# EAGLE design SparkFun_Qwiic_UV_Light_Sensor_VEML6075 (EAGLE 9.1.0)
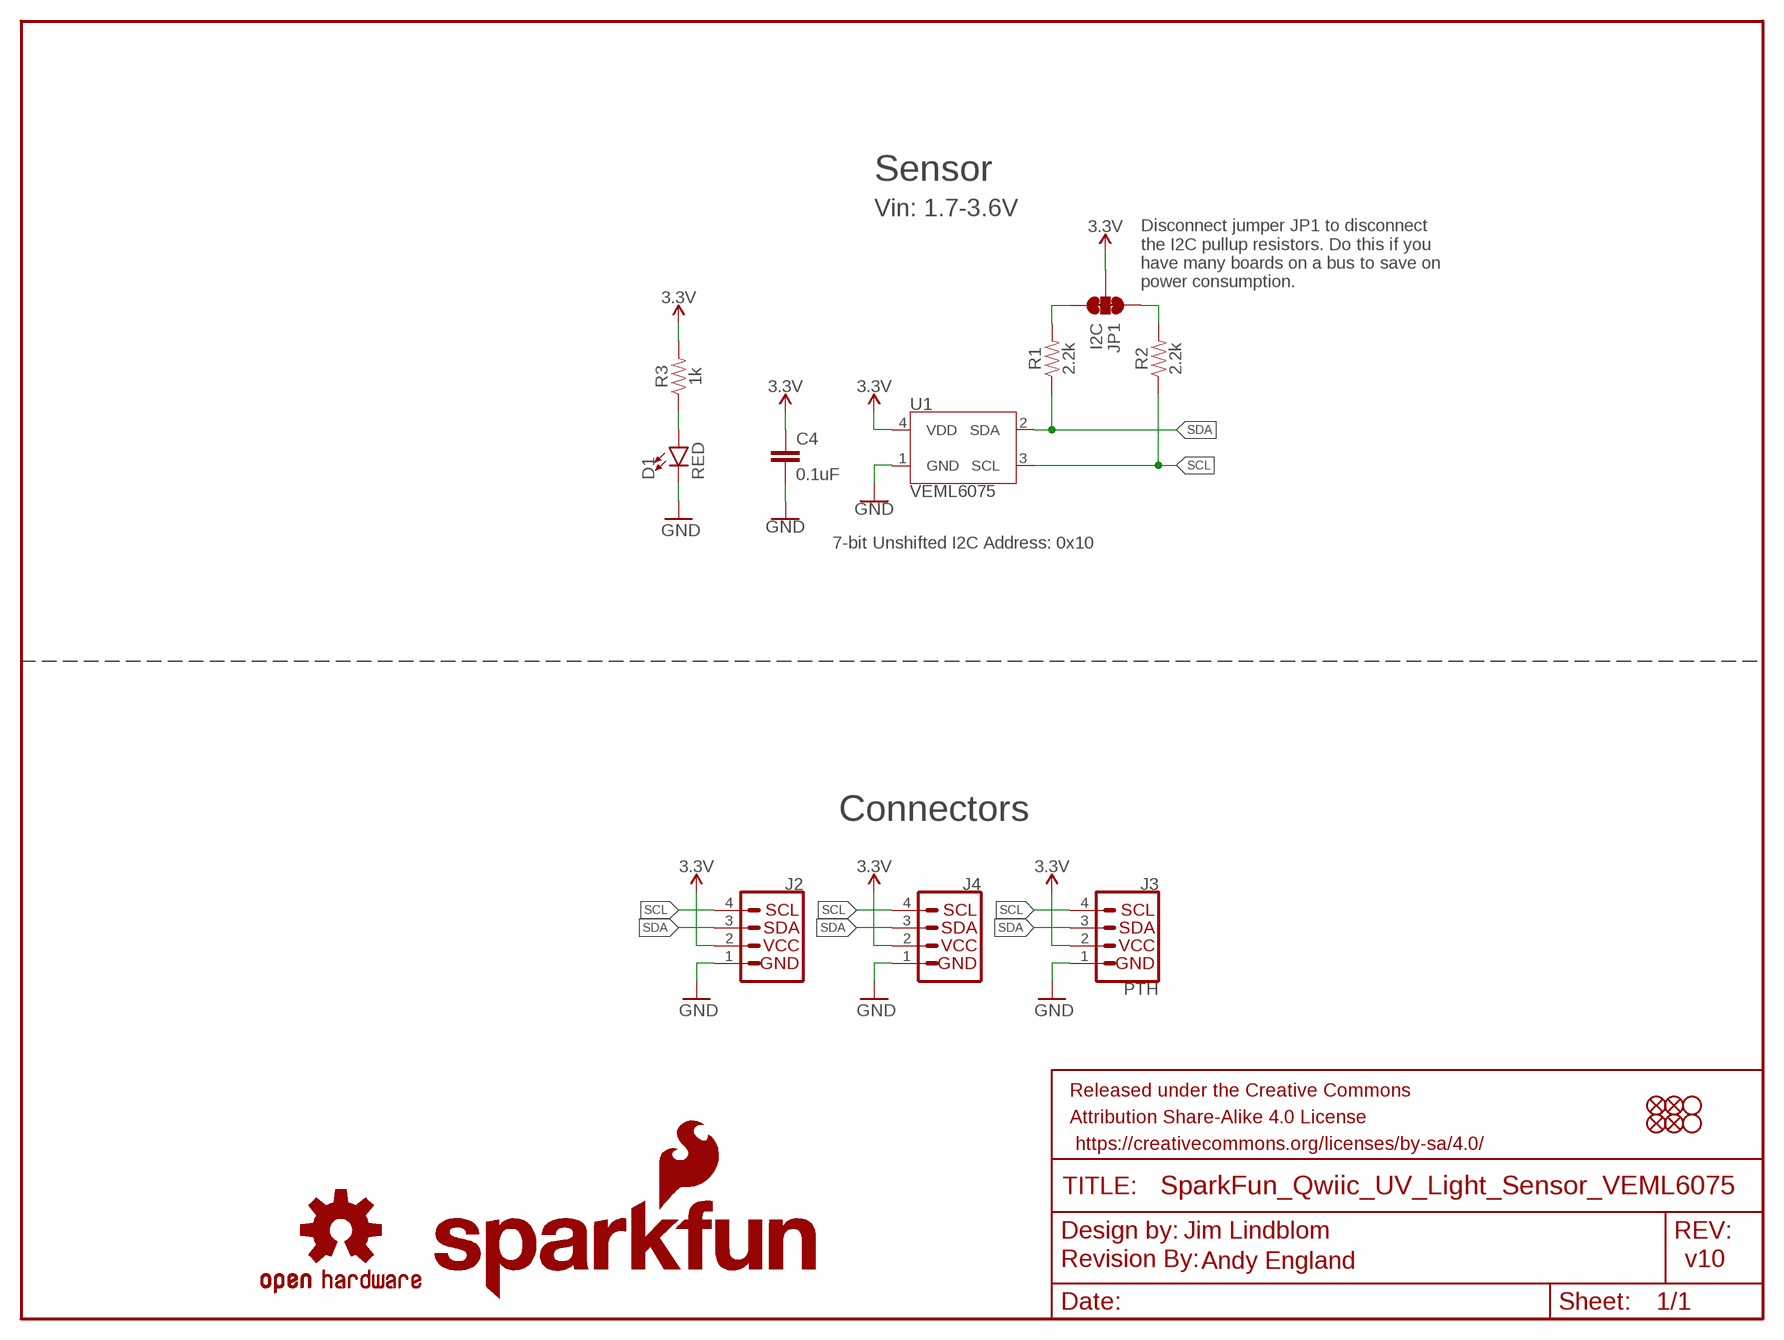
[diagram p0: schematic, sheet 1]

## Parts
C4  0.1uF  0.1UF-0603-25V-(+80/-20%)  [0603]
D1  RED  LED-RED0603  [LED-0603]
FRAME1  FRAME-LETTER  [CREATIVE_COMMONS]
J2  QWIIC_CONNECTORJS-1MM  [1X04_1MM_RA]
J3  PTH  I2C_STANDARD_NO_SILK  [1X04_NO_SILK]
J4  QWIIC_CONNECTORJS-1MM  [1X04_1MM_RA]
JP1  I2C  JUMPER-SMT_3_2-NC_TRACE_SILK  [SMT-JUMPER_3_2-NC_TRACE_SILK]
JP2  FIDUCIALUFIDUCIAL  [MICRO-FIDUCIAL]
JP3  STAND-OFF  [STAND-OFF]
JP4  STAND-OFF  [STAND-OFF]
JP5  FIDUCIALUFIDUCIAL  [MICRO-FIDUCIAL]
JP6  FIDUCIALUFIDUCIAL  [MICRO-FIDUCIAL]
JP7  FIDUCIALUFIDUCIAL  [MICRO-FIDUCIAL]
LOGO1  OSHW-LOGOMINI  [OSHW-LOGO-MINI]
LOGO2  REVISION  [REVISION]
R1  2.2k  2.2KOHM-0603-1/10W-1%  [0603]
R2  2.2k  2.2KOHM-0603-1/10W-1%  [0603]
R3  1k  1KOHM-0603-1/10W-1%  [0603]
U1  VEML6075  [VEML6075_A3OP]
U$1  SFE_LOGO_NAME_FLAME.1_INCH  [SFE_LOGO_NAME_FLAME_.1]
U$2  SFE_LOGO_NAME_FLAME.1_INCH  [SFE_LOGO_NAME_FLAME_.1]

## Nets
3.3V: C4.1 J2.2 J3.2(VCC) J4.2 JP1.2 R3.2 U1.4(VDD)
GND: C4.2 D1.C J2.1 J3.1(GND) J4.1 U1.1(GND)
N$3: D1.A R3.1
N$4: JP1.3 R1.2
N$5: JP1.1 R2.2
SCL: J2.4 J3.4(SCL) J4.4 R2.1 U1.3(SCL)
SDA: J2.3 J3.3(SDA) J4.3 R1.1 U1.2(SDA)

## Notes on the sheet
- Sensor
- Vin: 1.7-3.6V
- Disconnect jumper JP1 to disconnect 
  the I2C pullup resistors. Do this if you 
  have many boards on a bus to save on
  power consumption.
- 7-bit Unshifted I2C Address: 0x10
- Connectors
- Jim Lindblom
- Andy England | v10

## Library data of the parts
C4 = SparkFun-Capacitors:0.1UF: 0.1µF ceramic capacitors; PROD_ID: CAP-00810
D1 = SparkFun-LED:LED-RED: Red SMD LED; PROD_ID: DIO-00819
FRAME1 = SparkFun-Aesthetics:FRAME-LETTER: Schematic Frame - Letter
J2 J4 = SparkFun-Connectors:QWIIC_CONNECTOR: SparkFun I2C Standard Qwiic Connector An SMD 1mm pitch JST connector makes it easy and quick (get it? Qwiic?) to connect I2C devices to each other. The Qwiic system enables fast and solderless connection between popular platforms and various sensors and actuators. We carry 200mm, 100mm, 50mm, and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; PROD_ID: CONN-13694
J3 = SparkX:I2C_STANDARD: SparkFun I2C Standard Pinout Header SparkFun has standardized on a pinout for all I2C based sensor breakouts. This pinout allows I2C boards to be plugged directly into the headers on Arduino Uno compatible boards, and to be daisy chained easily. Example SparkFun Products: SparkFun Atmospheric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
JP1 = SparkFun-Jumpers:JUMPER-SMT_3_2-NC_TRACE: Normally closed trace jumper (2 of 2 connections) This jumper has a trace between all three pads so they are normally closed (NC). Use a razor knife to open the connection(s). For best results follow the IPC guidelines for cutting traces: Cutout at least 0.063 mm (0.005 in). Remove all loose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
JP2 JP5-JP7 = SparkFun:FIDUCIAL: Fiducial Alignment Points
JP3 JP4 = SparkFun:STAND-OFF: Stand Off
LOGO1 = SparkFun-Aesthetics:OSHW-LOGO: Open-Source Hardware (OSHW) Logo
LOGO2 = SparkFun-Aesthetics:REVISION: "Revision By" Text
R1 R2 = SparkFun-Resistors:2.2KOHM: 2.2kΩ resistor; PROD_ID: RES-08272
R3 = SparkFun-Resistors:1KOHM: 1kΩ resistor; PROD_ID: RES-07856
U1 = SparkFun-Sensors:VEML6075: Vishay VEML6075 UVA and UVB light sensor with I2C interface.; PROD_ID: IC-14149
U$1 U$2 = SparkFun-Aesthetics:SFE_LOGO_NAME_FLAME: SparkFun Font Logo w/ Flame

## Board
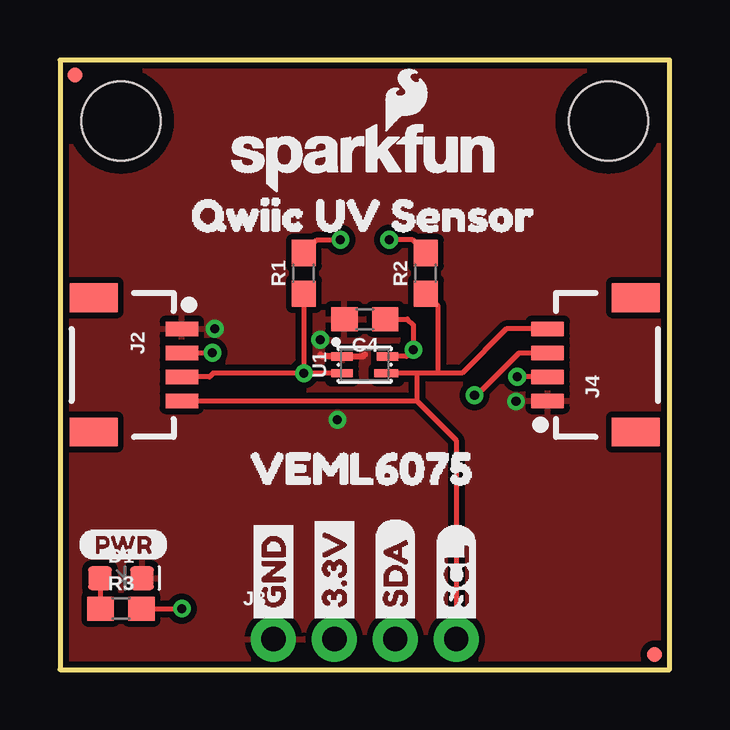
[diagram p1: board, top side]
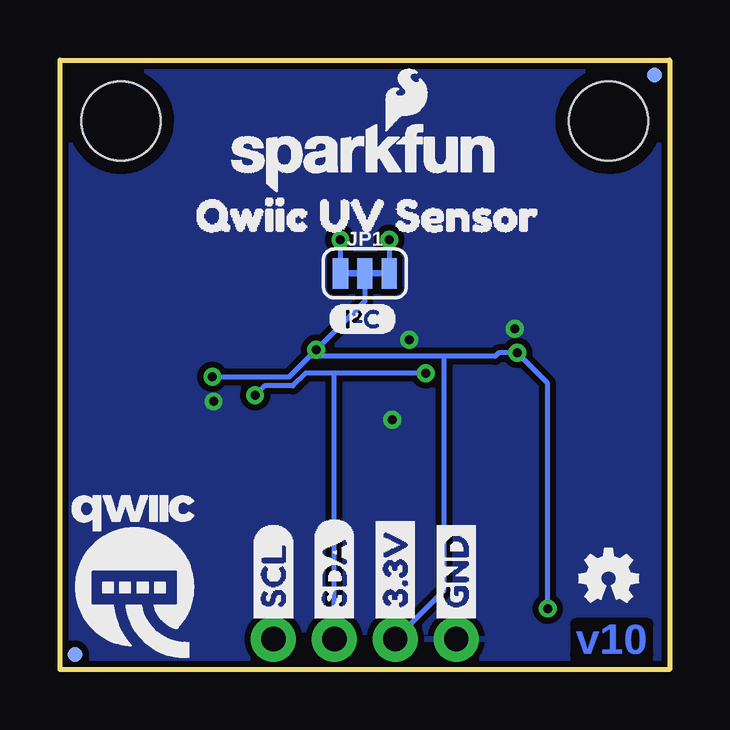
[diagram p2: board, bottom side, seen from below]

Size 25.4 x 25.4 mm. Coordinates in mm from the lower left corner, seen from the top.
Outline: 0,0 25.4,0 25.4,25.4 0,25.4 0,0
Copper layers (1*16): Top 0.035mm / dielectric 1.5mm / Bottom 0.035mm
Design rules "SparkFun-2-layer-TIGHT": minimum track width 7mil, minimum drill 15mil, track to track 7mil, track to pad 7mil, pad to pad 7mil, via to via 7mil, smd to smd 7mil, copper to edge 7mil, drill to drill 7mil, minimum pad ring 7mil, minimum via ring 7mil, stop-mask expansion 4mil, vias tented up to drill 25mil, thermal gap 10mil

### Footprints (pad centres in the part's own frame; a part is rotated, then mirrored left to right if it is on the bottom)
0603 = smd 1.1 x 1: 1 -0.85,0; 2 0.85,0
LED-0603 = smd 1 x 1: A -0.877,0; C 0.877,0
1X04_1MM_RA = smd 0.6 x 1.35: 1 -1.5,0; 2 -0.5,0; 3 0.5,0; 4 1.5,0 | smd 1.2 x 2: NC1 2.8,-3.675; NC2 -2.8,-3.675
1X04_NO_SILK = drill 1.016 pad 1.88: 1 0,0; 2 2.54,0; 3 5.08,0; 4 7.62,0
SMT-JUMPER_3_2-NC_TRACE_SILK = smd 0.635 x 1.27: 1 -1.016,0; 2 0,0; 3 1.016,0
MICRO-FIDUCIAL = smd 0.635 x 0.635: 1 0,0
STAND-OFF = hole 3.302: 0,0
VEML6075_A3OP = smd 0.9 x 0.35: 1 -0.95,0.35; 2 -0.95,-0.35; 4 0.95,0.35 | smd 1 x 0.35: 3 0.9,-0.35

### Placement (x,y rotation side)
C4  12.7,14.61 180 top
D1  2.54,3.81 0 top
FRAME1  not placed on the board
J2  5.08,12.7 270 top
J3  8.89,1.27 0 top
J4  20.32,12.7 90 top
JP1  12.7,16.51 0 bottom
JP2  24.77,0.64 0 bottom
JP3  2.54,22.86 0 top
JP4  22.86,22.86 90 top
JP5  24.77,0.64 0 top
JP6  0.64,24.77 0 top
JP7  0.64,24.77 0 bottom
LOGO1  2.54,3.81 0 bottom
LOGO2  not placed on the board
R1  10.16,16.51 90 top
R2  15.24,16.51 90 top
R3  2.54,2.54 0 top
U1  12.7,12.7 0 top
U$1  12.7,21.34 0 top
U$2  12.7,21.34 0 bottom
U$3  [QWIIC-LOGO-MEDIUM]  22.35,3.94 0 bottom
U$4  [GND1]  8.89,1.65 90 bottom
U$5  [QWIIC_UV_SENSOR1]  4.32,18.92 0 top
U$6  [_VEML60750]  6.35,8.38 0 top
U$7  [3#3V2]  11.43,1.65 90 bottom
U$8  [SDA8]  13.97,1.65 90 bottom
U$9  [SCL9]  16.51,1.65 90 bottom
U$10  [I_SUPER2_C-()-03]  14.22,14.61 0 bottom
U$11  [QWIIC_UV_SENSOR1]  20.9,18.92 0 bottom
U$16  [PWR-()-03]  0.76,5.21 0 top
U$21  [3#3V2]  11.43,1.65 90 top
U$22  [GND1]  8.89,1.65 90 top
U$26  [SCL9]  16.51,1.65 90 top
U$27  [SDA8]  13.97,1.65 90 top

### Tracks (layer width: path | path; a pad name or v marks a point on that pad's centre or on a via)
3.3V  (via drill 0.38)
  Top 0.203: J4.2 v19.05,12.2 | J2.2 v6.35,13.2 | R3.2 v5.08,2.54 | C4.1 14.48,14.61 14.72,14.36 v14.72,13.33 14.45,13.05 U1.4
  Bottom 0.203: v19.05,12.2 15.85,12.2 15,13.05 | 9.4,13.05 7.27,13.05 7.12,13.2 v6.35,13.2 5.08,11.93 v5.08,2.54 | 9.4,13.05 15,13.05 | JP1.2 12.7,15.35 v14.72,13.33 15,13.05 | J3.2 9.4,3.3 9.4,13.05
GND  (via drill 0.38)
  Top 0.254: 10.85,13.13 10.93,13.05 U1.1 12.62,13.05 12.7,13.13
  other vias: 11.56,10.41 6.45,14.2 19,11.18 10.85,13.74
  pour Top (isolate 0.254): 0,25.4 0,0 25.4,0 25.4,25.4
  pour Bottom (isolate 0.254): 25.4,25.4 25.4,0 0,0 0,25.4
N$3
  Top 0.203: R3.1 1.69,3.78 D1.A
N$4  (via drill 0.38)
  Top 0.203: R1.2 10.71,17.91 v11.68,17.91
  Bottom 0.203: v11.68,17.91 JP1.3
N$5  (via drill 0.38)
  Top 0.203: R2.2 14.69,17.91 v13.72,17.91
  Bottom 0.203: v13.72,17.91 JP1.1
SCL
  Top 0.203: 15.75,12.35 16.75,12.35 18.6,14.2 J4.4 | 15.75,12.35 14.86,12.35 | 14.86,12.35 U1.3 | R2.1 15.75,15.15 15.75,12.35 | J3.4 16.51,9.55 14.86,11.2 | J2.4 14.86,11.2 | 14.86,12.35 14.86,11.2
SDA  (via drill 0.38)
  Top 0.203: v10.16,12.35 6.38,12.35 6.23,12.2 J2.3 | R1.1 v10.16,12.35 | J4.3 19.13,13.2 17.36,11.43 v17.27,11.43 | U1.2 v10.16,12.35
  Bottom 0.203: v10.16,12.35 13.97,12.35 | 13.97,12.35 15.16,12.35 15.69,11.82 16.88,11.82 v17.27,11.43 | J3.3 13.97,12.35

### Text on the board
Bottom: v10
tDocu: Jim Lindblom | Andy England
